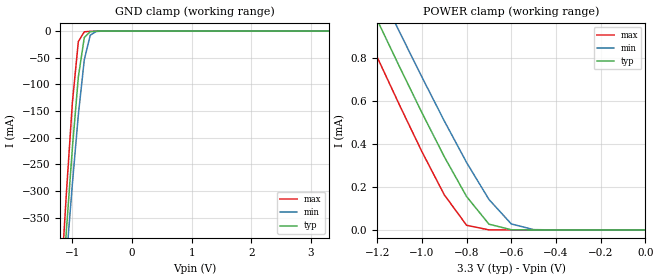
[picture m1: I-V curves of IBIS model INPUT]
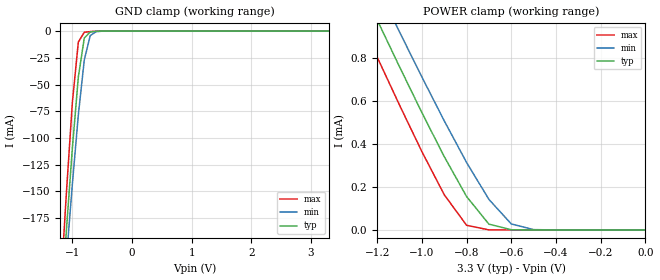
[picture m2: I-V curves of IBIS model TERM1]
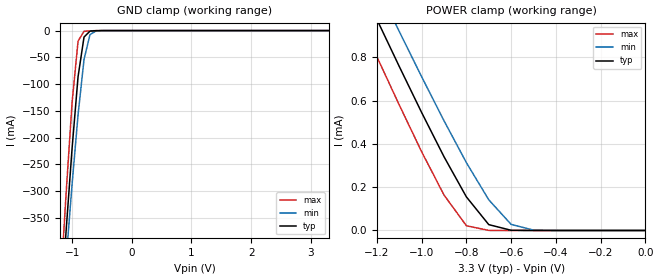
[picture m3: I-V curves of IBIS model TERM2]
|   PERICOM SEMICONDUCTOR CORP
|   IBIS Model of PI4MSD5V9545A
|   Product Family: 4MSD
|   TSSOP-20 (L) Package
[IBIS Ver] 3.2
[Comment char] |_char
[File Name] pi4msd5v9545a_l_33v.ibs
[File Rev] 1.0
[Source] File originated at Pericom Semiconductor Corp.
[Date] 09/07/17
[Disclaimer] (C) Copyright PERICOM Semiconductor Corporation
   All rights reserved
  Pericom Semiconductor Corporation hereby grants the user of
  this IBIS model a non-exclusive, nontransferable license to
  use this IBIS model under the following terms.
  This IBIS model is provided on an "AS IS" basis and Pericom
  makes absolutely no warranty with respect to the information
  contained herein. PERICOM DISCLAIMS AND CUSTOMER WAIVES ALL
  WARRANTIES, EXPRESSED OR IMPLIED, INCLUDING WARRANTIES OF
  MERCHANTABILITY OR FITNESS FOR A PARTICULAR PURPOSE. The
  entire risk as to quality and performance is with the customer.
  Accordingly, in no event shall the company be liable for any
  damages, whether in contract or tort, including any lost
  profits or other incidental, consequential, exemplary, or
  punitive damages arising out of the use or application of the
  IBIS model provided in this package. Further, Pericom reserves
  the right to make changes without notice to any product herein
  to improve reliability, function, or design. Pericom does not
  convey any license under patent rights or any other intellectual
  property rights, including those of third parties.
  The user is granted this license only to use the IBIS model
  and is not granted rights to sell, load, rent, lease or license
  the IBIS model in whole or in part, or in modified form to anyone
  other than user. User may modify the IBIS model to suit its specific
  application but rights to derivative works and such modifications
  shall belong to Pericom.
  Pericom is not obligated to provide maintenance or support
  for the licensed IBIS model.
  Contact Pericom at ATTN: APPLICATION ENGINEERING / IBIS MODELS
  2380 Bering Drive, San Jose, CA 95131
[Component] PI4MSD5V9545A
[Manufacturer] Pericom Semiconductor Corp.
[Package]
| variable   typ   min   max
R_pkg   0.03869ohm   0.03668ohm   0.04069ohm
L_pkg   2.64482nH   2.06962nH   3.22001nH
C_pkg   0.19279pF   0.15543pF   0.23014pF
[Pin] signal_name   model_name   R_pin   L_pin   C_pin
1   A0   INPUT   0.04069   3.22001nH   0.23014pF
2   A1   INPUT   0.03969   2.93241nH   0.21146pF
3   _RESET   INPUT   0.03869   2.64482nH   0.19279pF
4   _INT0   INPUT   0.03768   2.35722nH   0.17411pF
5   SD0   TERM1   0.03668   2.06962nH   0.15543pF
6   SC0   TERM1   0.03668   2.06962nH   0.15543pF
7   _INT1   INPUT   0.03768   2.35722nH   0.17411pF
8   SD1   TERM1   0.03869   2.64482nH   0.19279pF
9   SC1   TERM1   0.03969   2.93241nH   0.21146pF
10   GND   GND   0.04069   3.22001nH   0.23014pF
11   _INT2   INPUT   0.04069   3.22001nH   0.23014pF
12   SD2   TERM1   0.03969   2.93241nH   0.21146pF
13   SC2   TERM1   0.03869   2.64482nH   0.19279pF
14   _INT3   INPUT   0.03768   2.35722nH   0.17411pF
15   SD3   TERM1   0.03668   2.06962nH   0.15543pF
16   SC3   TERM1   0.03668   2.06962nH   0.15543pF
17   _INT   INPUT   0.03768   2.35722nH   0.17411pF
18   SCL   TERM2   0.03869   2.64482nH   0.19279pF
19   SDA   TERM2   0.03969   2.93241nH   0.21146pF
20   VCC   POWER   0.04069   3.22001nH   0.23014pF
[Series Switch Groups]
On 1 /
Off 2 3 4 /
[Series Pin Mapping]   pin_2   model_name  function_table_group
6   18   SWITCH1   1
5   19   SWITCH1   1
9   18   SWITCH1   2
8   19   SWITCH1   2
13   18   SWITCH1   3
12   19   SWITCH1   3
16   18   SWITCH1   4
15   19   SWITCH1   4
|   Model SWITCH1
[Model] SWITCH1
Model_type Series_switch
| variable   typ   min   max
C_comp   6.96pF   6.94pF   6.98pF
[Voltage Range]   3.3000V   3.0000V   3.6000V
[GND Clamp Reference]   0.0000V   0.0000V   0.0000V
[POWER Clamp Reference]   3.3000V   3.0000V   3.6000V
[Temperature Range]   25   85   -40
[On]
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[OFF]
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| Models and submodels in the file (4): INPUT (Input), SWITCH1 (Series_switch), TERM1 (Terminator), TERM2 (Terminator)
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|   Model INPUT
[Model] INPUT
Model_type Input
Vinl = 990mV
Vinh = 2.31V
| variable   typ   min   max
C_comp   4.38pF   4.37pF   4.39pF
[Voltage Range]   3.3000V   3.0000V   3.6000V
[GND Clamp Reference]   0.0000V   0.0000V   0.0000V
[POWER Clamp Reference]   3.3000V   3.0000V   3.6000V
[Temperature Range]   25   85   -40
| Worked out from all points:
|   GND clamp passes 1 mA (typ) near -0.70 V on its own axis
|   POWER clamp passes 1 mA (typ) near -1.21 V on its own axis
[GND Clamp]
| Voltage   I(typ)   I(min)   I(max)
-3.3V     -4.214A    -3.861A    -4.708A
-1.2V     -536.3mA   -573.9mA   -488.8mA
-1.1V     -373.8mA   -427.8mA   -304mA
-1V       -219.8mA   -287.2mA   -134.4mA
-900mV    -86.22mA   -157.4mA   -19.74mA
-800mV    -12.06mA   -53.77mA   -1.311mA
-700mV    -1.032mA   -7.522mA   -526.9uA
-600mV    -210.6uA   -734.5uA   -129.9uA
3.3V      125.8pA    2.663nA    123.3pA
[POWER Clamp]   |Note: Vtable = Vcc - Voutput
| Voltage   I(typ)   I(min)   I(max)
-3.3V     5.749mA    5.788mA    5.712mA
-1.3V     1.195mA    1.347mA    1.029mA
-1.2V     974.9uA    1.132mA    802.5uA
-1.1V     757.6uA    919.3uA    579.7uA
-1V       544.9uA    710.2uA    363.8uA
-900mV    340.5uA    506.6uA    163.7uA
-800mV    155.1uA    313.2uA    21.83uA
-700mV    27.01uA    141.6uA    235.8nA
-600mV    852.5nA    28.01uA    1.791nA
-500mV    17.74nA    1.596uA    170.4pA
0V        125.8pA    153.2pA    136.8pA
|   Model TERM1
[Model] TERM1
Model_type Terminator
| variable   typ   min   max
C_comp   2.58pF   2.57pF   2.59pF
[Voltage Range]   3.3000V   3.0000V   3.6000V
[GND Clamp Reference]   0.0000V   0.0000V   0.0000V
[POWER Clamp Reference]   3.3000V   3.0000V   3.6000V
[Temperature Range]   25   85   -40
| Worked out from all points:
|   GND clamp passes 1 mA (typ) near -0.70 V on its own axis
|   POWER clamp passes 1 mA (typ) near -1.21 V on its own axis
[GND Clamp]
| Voltage   I(typ)   I(min)   I(max)
-3.3V     -2.1A      -1.924A    -2.346A
-1.2V     -267.2mA   -286mA     -243.4mA
-1.1V     -186.2mA   -213.2mA   -151.2mA
-1V       -109.4mA   -143.1mA   -66.79mA
-900mV    -42.98mA   -78.43mA   -10.22mA
-800mV    -6.45mA    -26.94mA   -1.105mA
-700mV    -805uA     -4.15mA    -477.3uA
-600mV    -185.9uA   -544.9uA   -115.7uA
3.3V      68.73pA    2.569nA    67.15pA
[POWER Clamp]   |Note: Vtable = Vcc - Voutput
| Voltage   I(typ)   I(min)   I(max)
-3.3V     5.749mA    5.788mA    5.712mA
-1.3V     1.195mA    1.347mA    1.029mA
-1.2V     974.9uA    1.132mA    802.5uA
-1.1V     757.6uA    919.3uA    579.7uA
-1V       544.9uA    710.2uA    363.8uA
-900mV    340.5uA    506.6uA    163.7uA
-800mV    155.1uA    313.2uA    21.83uA
-700mV    27.01uA    141.6uA    235.7nA
-600mV    852.4nA    28.01uA    1.717nA
-500mV    17.67nA    1.596uA    99.08pA
0V        68.73pA    67.71pA    74.93pA
|   Model TERM2
[Model] TERM2
Model_type Terminator
| variable   typ   min   max
C_comp   4.38pF   4.37pF   4.39pF
[Voltage Range]   3.3000V   3.0000V   3.6000V
[GND Clamp Reference]   0.0000V   0.0000V   0.0000V
[POWER Clamp Reference]   3.3000V   3.0000V   3.6000V
[Temperature Range]   25   85   -40
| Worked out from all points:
|   GND clamp passes 1 mA (typ) near -0.70 V on its own axis
|   POWER clamp passes 1 mA (typ) near -1.21 V on its own axis
[GND Clamp]
| Voltage   I(typ)   I(min)   I(max)
-3.3V     -4.214A    -3.861A    -4.708A
-1.2V     -536.3mA   -573.9mA   -488.8mA
-1.1V     -373.8mA   -427.8mA   -304mA
-1V       -219.8mA   -287.2mA   -134.4mA
-900mV    -86.22mA   -157.4mA   -19.74mA
-800mV    -12.06mA   -53.77mA   -1.311mA
-700mV    -1.032mA   -7.522mA   -526.9uA
-600mV    -210.6uA   -734.5uA   -129.9uA
3.3V      125.8pA    2.663nA    123.3pA
[POWER Clamp]   |Note: Vtable = Vcc - Voutput
| Voltage   I(typ)   I(min)   I(max)
-3.3V     5.749mA    5.788mA    5.712mA
-1.3V     1.195mA    1.347mA    1.029mA
-1.2V     974.9uA    1.132mA    802.5uA
-1.1V     757.6uA    919.3uA    579.7uA
-1V       544.9uA    710.2uA    363.8uA
-900mV    340.5uA    506.6uA    163.7uA
-800mV    155.1uA    313.2uA    21.83uA
-700mV    27.01uA    141.6uA    235.8nA
-600mV    852.5nA    28.01uA    1.791nA
-500mV    17.74nA    1.596uA    170.4pA
0V        125.8pA    153.2pA    136.8pA
